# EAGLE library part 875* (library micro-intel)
MICROCOMPUTER/PERIPHERAL DEVICE
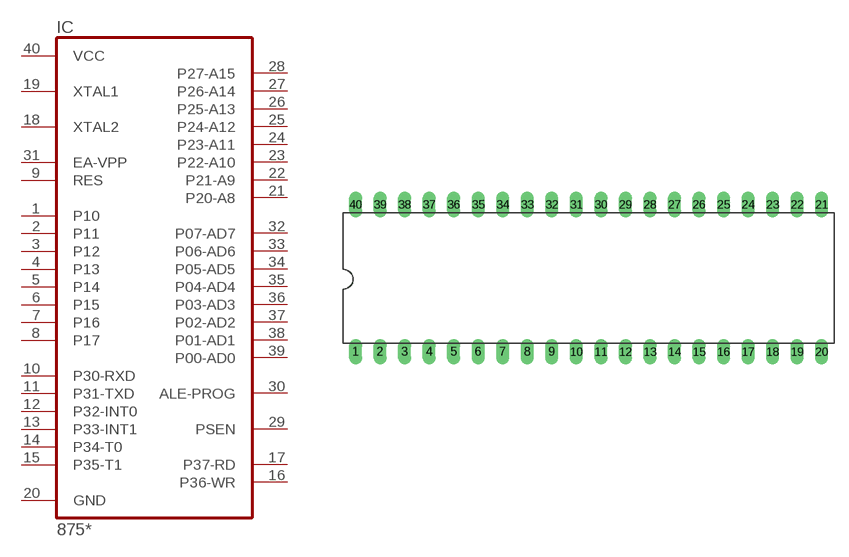
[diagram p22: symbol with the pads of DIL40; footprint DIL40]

Designator prefix IC

## 8751P (OC_FARNELL: unknown; OC_NEWARK: unknown), 8752P (OC_FARNELL: unknown; OC_NEWARK: unknown)  [DIL40]
1  P10
2  P11
3  P12
4  P13
5  P14
6  P15
7  P16
8  P17
9  RES  in
10  P30-RXD
11  P31-TXD
12  P32-INT0
13  P33-INT1
14  P34-T0
15  P35-T1
16  P36-WR
17  P37-RD
18  XTAL2  in
19  XTAL1  in
20  GND  pwr
21  P20-A8
22  P21-A9
23  P22-A10
24  P23-A11
25  P24-A12
26  P25-A13
27  P26-A14
28  P27-A15
29  PSEN  out
30  ALE-PROG  out
31  EA-VPP  in
32  P07-AD7
33  P06-AD6
34  P05-AD5
35  P04-AD4
36  P03-AD3
37  P02-AD2
38  P01-AD1
39  P00-AD0
40  VCC  pwr

## Footprint DIL40 (pad centres in mm)
Dual In Line Package
drill 0.813 long: 1 -24.13,-7.62; 2 -21.59,-7.62; 3 -19.05,-7.62; 4 -16.51,-7.62; 5 -13.97,-7.62; 6 -11.43,-7.62; 7 -8.89,-7.62; 8 -6.35,-7.62; 9 -3.81,-7.62; 10 -1.27,-7.62; 11 1.27,-7.62; 12 3.81,-7.62; 13 6.35,-7.62; 14 8.89,-7.62; 15 11.43,-7.62; 16 13.97,-7.62; 17 16.51,-7.62; 18 19.05,-7.62; 19 21.59,-7.62; 20 24.13,-7.62; 21 24.13,7.62; 22 21.59,7.62; 23 19.05,7.62; 24 16.51,7.62; 25 13.97,7.62; 26 11.43,7.62; 27 8.89,7.62; 28 6.35,7.62; 29 3.81,7.62; 30 1.27,7.62; 31 -1.27,7.62; 32 -3.81,7.62; 33 -6.35,7.62; 34 -8.89,7.62; 35 -11.43,7.62; 36 -13.97,7.62; 37 -16.51,7.62; 38 -19.05,7.62; 39 -21.59,7.62; 40 -24.13,7.62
